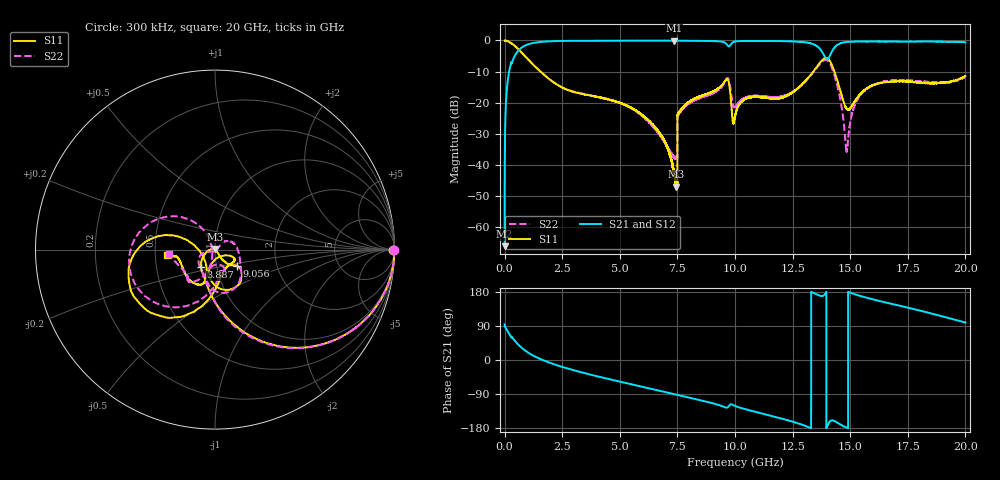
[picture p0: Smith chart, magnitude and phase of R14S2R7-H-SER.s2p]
!{R14S2R7}
!Johanson Technology Inc.
!www.johansontechnology.com
!Test Board Conditions:
!Substrate Type  RO4350B
!Substrate Thickness  20 mil
!Substrate Dk  3.66
!TL Type: GCPW
!TL Trace Width  36 mil
!TL Gap  12 mil
!Electrode orientation  Horizontal
!DUT TOPOLOGY	SERIES
!Mounting Pad LxW  26x36 mil
! Created Wed Nov 25 17:33:21 2020
! 2 Port Network Data from SP1.SP block
! freq  magS11  angS11  magS21  angS21  magS12  angS12  magS22  angS22
# khz S ma R 50
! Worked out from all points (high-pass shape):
!   20001 points, 300 kHz to 20 GHz, reference 50 ohm
!   highest |S21| = -0.04 dB at 7.358 GHz (marker M1); lowest = -66.2 dB at 300 kHz (marker M2)
!   |S21| within 3 dB of the highest: 624.4 MHz to 13.72 GHz (13.1 GHz wide, 183 % of centre); 14.25 GHz to end of sweep
!   lowest |S11| = -47.0 dB at 7.427 GHz (marker M3), VSWR 1.01, Z = 49.9 + j0.424 ohm
!   |S11| at or under -10 dB: 1.558 GHz to 13.4 GHz (11.84 GHz wide, 158 % of centre); 14.32 GHz to end of sweep
!   |S22| runs from -38.1 to 0.0 dB; largest |S21 - S12| = 0.019
!   S11 on the Smith chart (normalised r, x): 300 kHz: open; 3.887 GHz: 0.84, -0.17; 9.056 GHz: 1.25, -0.23; 20 GHz: 0.58, -0.04
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300  0.9923 -0.2  0.0004925 94.2  0.0004478 87.2  0.9969 -0.1
127300  0.9759 -13.5  0.2106 76.3  0.2115 76.3  0.9771 -13.6
453300  0.8129 -39.7  0.5778 49.9  0.5791 49.9  0.8122 -39.9
1406300  0.356 -83.0  0.9306 6.6  0.9313 6.5  0.3578 -83.5
3334300  0.139 -122.0  0.9864 -32.4  0.9867 -32.5  0.1404 -121.6
3887300  0.1264 -128.5  0.9872 -41.0  0.9884 -40.9  0.1272 -132.2
6667300  0.03467 -173.0  0.9931 -80.4  0.9933 -80.4  0.03256 -159.2
7358300  0.006955 139.1  0.9951 -90.1  0.9941 -90.1  0.01304 -110.9
7427300  0.004464 107.7  0.9922 -91.1  0.9936 -91.1  0.01296 -96.7
7600300  0.07231 -52.6  0.99 -93.5  0.9901 -93.5  0.06893 40.7
9056300  0.1512 -36.8  0.9783 -114.6  0.979 -114.6  0.1425 -16.9
9663300  0.2398 -65.2  0.8466 -125.7  0.8473 -125.6  0.2458 -68.5
1.00003e7  0.06014 -33.2  0.9598 -121.1  0.9611 -121.1  0.08491 -78.5
1.04353e7  0.1146 -23.3  0.9787 -129.7  0.9786 -129.7  0.1192 -63.8
1.33343e7  0.2951 -99.4  0.89 179.2  0.8929 179.1  0.2876 -105.7
1.37763e7  0.4763 -128.6  0.6569 168.7  0.6602 168.1  0.4536 -140.9
1.41373e7  0.4549 -176.3  0.5852 -160.7  0.5855 -161.2  0.4123 162.5
1.45093e7  0.1856 160.4  0.8775 -168.0  0.879 -168.1  0.1458 122.2
1.48503e7  0.07915 -163.5  0.9451 -178.5  0.945 -178.5  0.01637 -166.5
1.53883e7  0.1305 -110.8  0.9606 170.0  0.9641 169.8  0.125 -108.4
1.66673e7  0.2139 -115.7  0.9627 149.9  0.9553 149.8  0.2267 -126.5
2e7  0.2682 -173.3  0.9381 98.9  0.9379 99.1  0.26 -174.4
